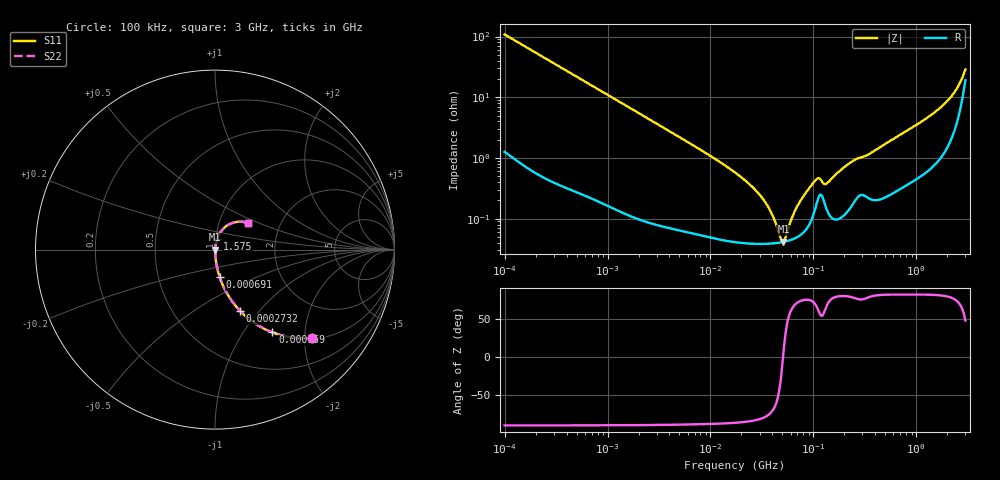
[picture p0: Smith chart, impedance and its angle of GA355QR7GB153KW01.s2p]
!Murata Part Number: GA355QR7GB153KW01
!These Parameters are Measured in Series Mode Connection
!Data Generated on Jun 19, 2026
!  o--ll--o
!Port1  Port2
!  o------o
!Operation Temp=25[degC], DC Bias Voltage=0[V]
!Freq. Start=100[kHz] Stop=3[GHz] 401[Steps]
# Hz S RI R 50
!Freq.(Hz) S11(Real) S11(Imag) S21(Real) S21(Imag) S12(Real) S12(Imag) S22(Real) S22(Imag)
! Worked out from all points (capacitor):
!   401 points, 100 kHz to 3 GHz, reference 50 ohm
!   read as one part in series: C = 14.7 nF near 105.3 kHz
!   lowest |Z| = 41.5 mohm at 51.13 MHz (marker M1)
!   series resonance near 50.7 MHz, so ESL is about 670 pH
!   S11 on the Smith chart (normalised r, x): 100 kHz: 1.03, -2.16; 159 kHz: 1.01, -1.36; 273.2 kHz: 1.01, -0.80; 691 kHz: 1.00, -0.32; 1.575 GHz: 1.02, +0.12; 3 GHz: 1.38, +0.43
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100000  0.5388 -0.4927  0.4612 0.4927  0.4612 0.4927  0.5388 -0.4927
159027  0.3194 -0.461  0.6806 0.461  0.6806 0.461  0.3194 -0.461
273224  0.1394 -0.3411  0.8606 0.3411  0.8606 0.3411  0.1394 -0.3411
562235  0.0386 -0.1863  0.9614 0.1863  0.9614 0.1863  0.0386 -0.1863
690972  0.0265 -0.1538  0.9735 0.1538  0.9735 0.1538  0.0265 -0.1538
3161081  0.00198 -0.0348  0.998 0.0348  0.998 0.0348  0.00198 -0.0348
1.77727e7  0.000438 -0.00556  0.9996 0.00556  0.9996 0.00556  0.000438 -0.00556
2.549486e7  0.000396 -0.00332  0.9996 0.00332  0.9996 0.00332  0.000396 -0.00332
3.298988e7  0.000387 -0.00199  0.9996 0.00199  0.9996 0.00199  0.000387 -0.00199
3.951212e7  0.000391 -0.00114  0.9996 0.00114  0.9996 0.00114  0.000391 -0.00114
4.855934e7  0.000407 -0.000196  0.9996 0.000196  0.9996 0.000196  0.000407 -0.000196
5.112795e7  0.000413 3.83e-05  0.9996 -3.83e-05  0.9996 -3.83e-05  0.000413 3.83e-05
5.383243e7  0.000421 0.000274  0.9996 -0.000274  0.9996 -0.000274  0.000421 0.000274
6.788584e7  0.000485 0.00138  0.9995 -0.00138  0.9995 -0.00138  0.000485 0.00138
9.738194e7  0.00103 0.00354  0.999 -0.00354  0.999 -0.00354  0.00103 0.00354
1.107752e8  0.0021 0.0041  0.9979 -0.0041  0.9979 -0.0041  0.0021 0.0041
1.361397e8  0.00137 0.00357  0.9986 -0.00357  0.9986 -0.00357  0.00137 0.00357
2.339019e8  0.00166 0.00842  0.9983 -0.00842  0.9983 -0.00842  0.00166 0.00842
5.475153e8  0.00276 0.0185  0.9972 -0.0185  0.9972 -0.0185  0.00276 0.0185
1.575075e9  0.0116 0.0581  0.9884 -0.0581  0.9884 -0.0581  0.0116 0.0581
2.441062e9  0.0481 0.1184  0.9519 -0.1184  0.9519 -0.1184  0.0481 0.1184
3e9  0.1864 0.147  0.8136 -0.147  0.8136 -0.147  0.1864 0.147
